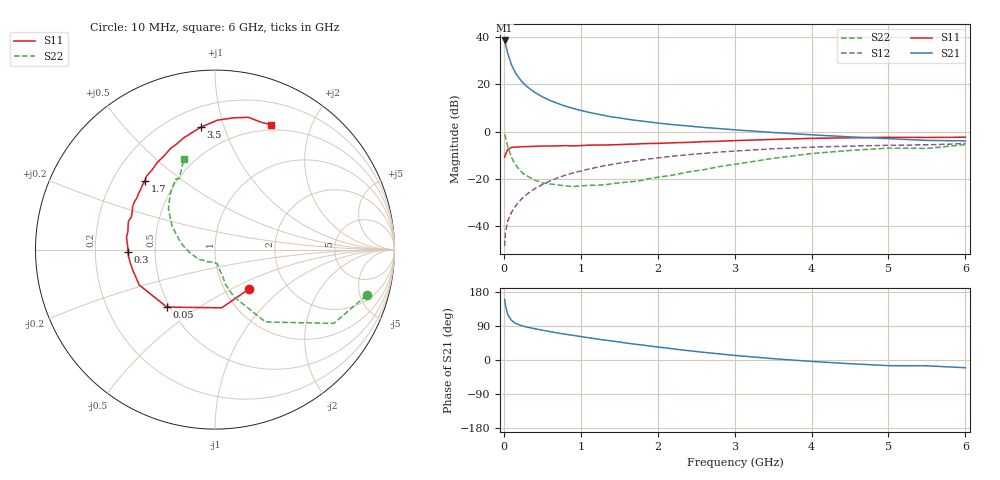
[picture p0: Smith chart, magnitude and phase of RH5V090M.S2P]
! SIEMENS Small Signal Semiconductors
! BFR106
! Si NPN RF Bipolar Junction Transistor in SOT23
! VCE = 5 V  IC = 90 mA
! Common Emitter S-Parameters:  August  1996
# GHz  S  MA  R  50
!  f  S11  S21  S12  S22
! GHz  MAG  ANG  MAG  ANG  MAG  ANG  MAG  ANG
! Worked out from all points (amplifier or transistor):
!   36 points, 10 MHz to 6 GHz, reference 50 ohm
!   highest |S21| = 38.6 dB at 10 MHz (marker M1)
!   |S21| within 3 dB of that: start of sweep to 32.8 MHz
!   unconditionally stable (mu >= 1): 184.3 MHz to 2.413 GHz
!   at 250 MHz: K = 1.05, MAG = 22.9 dB, |S12| = -27.9 dB
!   at 1.4 GHz: K = 1.07, MAG = 8.5 dB, |S12| = -13.9 dB
!   at 6 GHz: K = 0.99, MSG = 0.6 dB, |S12| = -5.0 dB
!   S11 on the Smith chart (normalised r, x): 10 MHz: 1.30, -0.62; 50 MHz: 0.48, -0.37; 300 MHz: 0.35, -0.01; 1.7 GHz: 0.34, +0.37; 3.5 GHz: 0.32, +0.84; 6 GHz: 0.44, +1.45
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0.01  0.2901 -49.0  84.69 160.5  0.0038 78.8  0.8819 -16.8
0.02  0.3265 -83.4  73.55 145.6  0.0073 72.1  0.7794 -31.8
0.05  0.4176 -129.9  45.56 120.1  0.0128 61.5  0.4919 -55.1
0.1  0.4661 -155.0  25.79 104.4  0.0198 66.1  0.2845 -68.0
0.15  0.4719 -165.7  17.59 97.0  0.0266 68.6  0.2017 -73.4
0.2  0.4781 -171.3  13.39 92.8  0.0333 71.1  0.1593 -73.7
0.25  0.4833 -175.5  10.73 89.4  0.0405 72.2  0.1301 -75.6
0.3  0.4836 -178.4  8.983 86.9  0.0479 73.4  0.1168 -77.1
0.4  0.4891 176.2  6.799 82.7  0.0621 74.0  0.0945 -79.1
0.5  0.4979 172.3  5.457 78.7  0.0763 73.6  0.0829 -80.3
0.6  0.4955 168.2  4.574 75.0  0.0908 72.8  0.0783 -83.2
0.7  0.5016 164.8  3.95 71.2  0.1055 72.0  0.0752 -87.9
0.8  0.5075 161.8  3.465 68.1  0.1199 70.6  0.0714 -92.2
1.1  0.5181 152.4  2.576 58.8  0.1618 66.8  0.0732 -106.0
1.4  0.5283 143.8  2.063 50.3  0.2019 62.4  0.0789 -121.3
1.7  0.546 135.7  1.747 41.8  0.2411 58.1  0.0888 -138.7
2.2  0.5819 123.6  1.406 29.4  0.3034 50.3  0.1208 -162.8
2.8  0.6261 109.9  1.162 16.2  0.3691 40.9  0.1827 171.8
3.5  0.6861 96.7  0.96 3.5  0.435 30.4  0.2729 151.3
4.5  0.7419 81.8  0.776 -9.8  0.4948 15.7  0.4008 128.3
5.5  0.7547 69.8  0.653 -15.4  0.5261 6.2  0.443 116.8
6  0.7625 65.9  0.639 -20.4  0.5615 -0.9  0.5337 108.9
